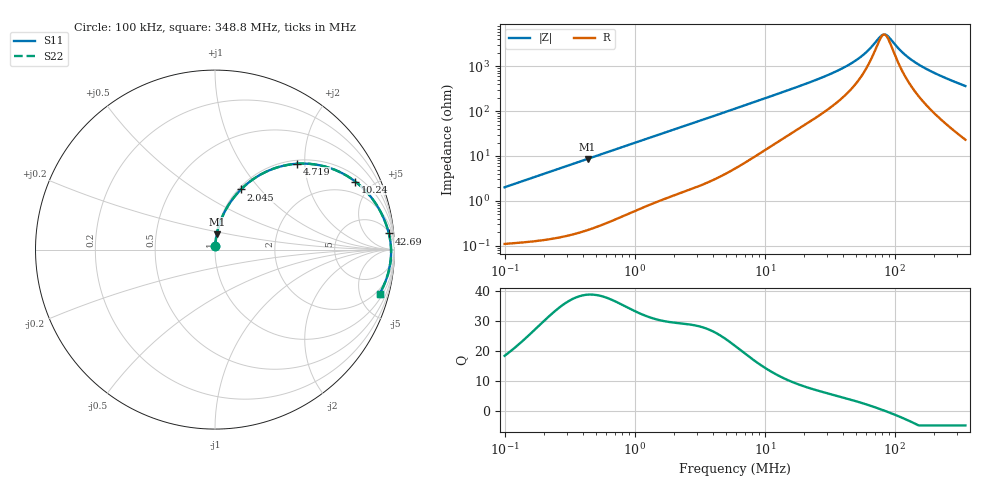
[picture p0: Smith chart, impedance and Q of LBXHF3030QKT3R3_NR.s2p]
! LBXHF3030QKT3R3_NR  S-PARAMETER MODEL  ( General Type )
! Model Generated by TAIYO YUDEN Corporation (http://www.ty-top.com)
! Version 1.0
! TAIYO YUDEN Control No. 210113NI43SB-FBB
! Copyright(c) 2021 TAIYO YUDEN CO.,LTD. All Rights Reserved.
! Product Description (link to TY-COMPAS)
! https://ds.yuden.co.jp/TYCOMPAS/or/detail?pn=LBXHF3030QKT3R3MNR&u=M
! Products Name : Inductors
! Characteristics :
!  Inductance : 3.3 uH , SRF(min) : 55 MHz , DC Resistance(max) : 0.096 Ohm
!  Rated Current : Saturation :1200 mA , Temp Rise : 1200 mA
!  Case Size : 3.0 x 3.0 / 0.118 x 0.118 [mm/inch] , Thickness : 1.5 / 0.059 [mm/inch]
!  (Conditions: Temperature = 25 degC , DC Bias Current/Voltage = 0A / 0V)
! External Node Assignments :
!  1  o---GGG---o  2
! GND o---------o GND
! Frequency Range : 0.1MHz  -  348.750116MHz  [ 402 STEP ]
# MHz S RI R 50
! Freq[MHz].  S11 Real  S11 Imag  S21 Real  S21 Imag  S12 Real  S12 Imag  S22 Real  S22 Imag
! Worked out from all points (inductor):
!   401 points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, 100 kHz to 348.8 MHz, reference 50 ohm
!   read as one part in series: L = 3.19 uH near 104.2 kHz
!   highest Q = 38.9 at 434.2 kHz (marker M1), where L = 3.17 uH
!   self-resonance near 82.71 MHz
!   S11 on the Smith chart (normalised r, x): 100 kHz: 1.00, +0.04; 2.045 MHz: 1.03, +0.79; 4.719 MHz: 1.07, +1.82; 10.24 MHz: 1.28, +3.96; 42.69 MHz: 6, +20; 348.8 MHz: 1.46, -7.29
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0.1  0.00149 0.02  0.9985 -0.02  0.9985 -0.02  0.00149 0.02
0.392077  0.00804 0.0773  0.992 -0.0773  0.992 -0.0773  0.00804 0.0773
0.434163  0.00957 0.0854  0.9904 -0.0854  0.9904 -0.0854  0.00957 0.0854
0.833784  0.0307 0.159  0.9693 -0.159  0.9693 -0.159  0.0307 0.159
1.537242  0.0903 0.2706  0.9097 -0.2706  0.9097 -0.2706  0.0903 0.2706
2.045174  0.1448 0.3353  0.8552 -0.3353  0.8552 -0.3353  0.1448 0.3353
3.013004  0.2607 0.4218  0.7393 -0.4218  0.7393 -0.4218  0.2607 0.4218
4.71887  0.4552 0.4782  0.5448 -0.4782  0.5448 -0.4782  0.4552 0.4782
5.905507  0.5625 0.4736  0.4375 -0.4736  0.4375 -0.4736  0.5625 0.4736
10.24181  0.7815 0.3793  0.2185 -0.3793  0.2185 -0.3793  0.7815 0.3793
14.78393  0.8705 0.2909  0.1295 -0.2909  0.1295 -0.2909  0.8705 0.2909
23.15412  0.9313 0.1932  0.0687 -0.1932  0.0687 -0.1932  0.9313 0.1932
32.74803  0.9567 0.131  0.0433 -0.131  0.0433 -0.131  0.9567 0.131
42.68909  0.9687 0.0898  0.0313 -0.0898  0.0313 -0.0898  0.9687 0.0898
57.96438  0.977 0.0469  0.023 -0.0469  0.023 -0.0469  0.977 0.0469
78.70557  0.9808 0.00649  0.0192 -0.00649  0.0192 -0.00649  0.9808 0.00649
83.67088  0.9811 -0.00151  0.0189 0.00151  0.0189 0.00151  0.9811 -0.00151
90.78195  0.9812 -0.0122  0.0188 0.0122  0.0188 0.0122  0.9812 -0.0122
115.9511  0.9799 -0.0453  0.0201 0.0453  0.0201 0.0453  0.9799 -0.0453
148.0984  0.9757 -0.0809  0.0243 0.0809  0.0243 0.0809  0.9757 -0.0809
218.1824  0.9605 -0.1462  0.0395 0.1462  0.0395 0.1462  0.9605 -0.1462
348.7501  0.9169 -0.2462  0.0831 0.2462  0.0831 0.2462  0.9169 -0.2462
